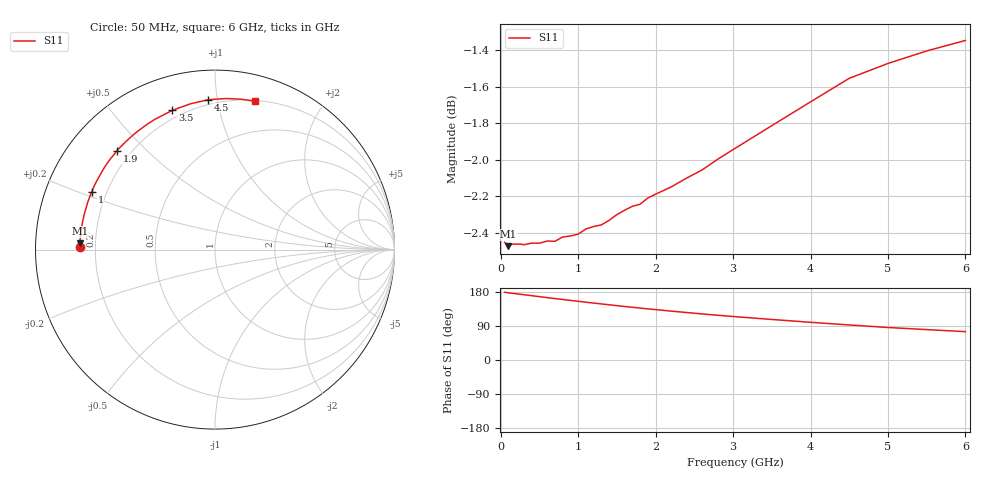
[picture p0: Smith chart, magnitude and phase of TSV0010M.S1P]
! SIEMENS Small Signal Semiconductors
! BAT14-03W
! Si Schottky Diode in SOD323
! IF = 10 mA
! S-Parameters:  November  1995
# GHz  S  MA  R  50
!  f  S11
! GHz  MAG  ANG
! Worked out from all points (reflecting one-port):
!   34 points, 50 MHz to 6 GHz, reference 50 ohm
!   lowest |S11| = -2.5 dB at 100 MHz (marker M1), VSWR 7.08, Z = 7.07 + j1.15 ohm
!   phase of S11 starts at 179 deg and turns -104 deg over the sweep
!   S11 on the Smith chart (normalised r, x): 50 MHz: 0.14, +0.01; 1 GHz: 0.14, +0.22; 1.9 GHz: 0.15, +0.41; 3.5 GHz: 0.16, +0.73; 4.5 GHz: 0.17, +0.94; 6 GHz: 0.21, +1.29
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0.05  0.7542 178.7
0.1  0.7523 177.3
0.15  0.7533 176.0
0.2  0.7533 174.8
0.3  0.753 172.2
0.4  0.7538 169.7
0.6  0.7548 164.6
0.8  0.7567 159.7
1  0.7581 154.9
1.1  0.7605 152.6
1.2  0.7617 150.2
1.3  0.7625 148.0
1.5  0.7674 143.4
1.6  0.7695 141.2
1.7  0.7714 139.1
1.9  0.7755 134.9
2  0.7773 133.0
2.2  0.7809 129.0
2.4  0.7852 125.3
2.6  0.7893 121.6
2.8  0.7945 118.1
3  0.7994 114.8
3.5  0.8115 107.0
4  0.8238 99.5
4.5  0.8361 92.5
5  0.8439 85.8
5.5  0.8506 80.2
6  0.8562 74.8
